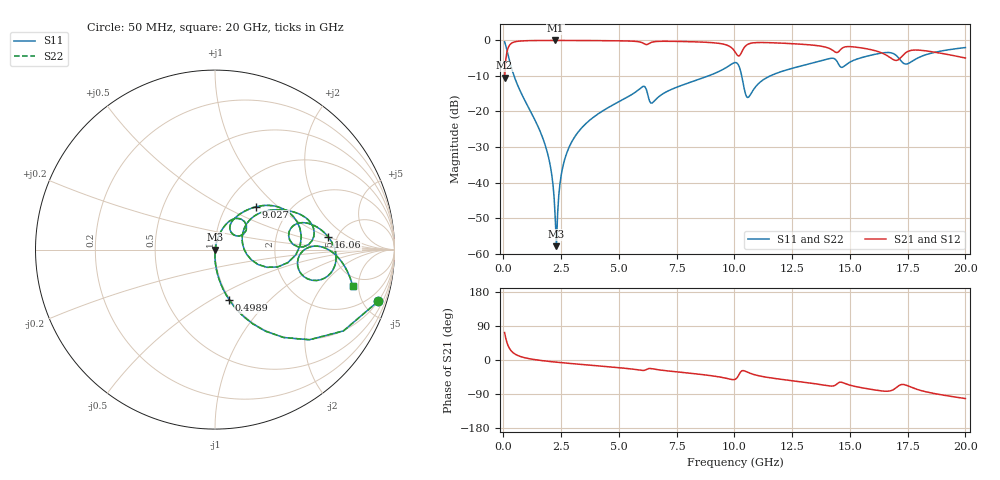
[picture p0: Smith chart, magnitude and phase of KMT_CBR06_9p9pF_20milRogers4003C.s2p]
! Data measured by Modelithics Inc. support@modelithics.com 813-866-6335
! KEMET CBR0603 9.9pF, Pad Width= 0.851mm, Pad Length= 0.64mm, Pad Gap= 0.62mm, 20mil Rogers 4003C substrate Data, January 2022
# hz S ma R 50
! 2 Port Network Data from SP1.SP block
! freq  magS11  angS11  magS21  angS21  magS12  angS12  magS22  angS22
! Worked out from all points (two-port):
!   401 points, 50 MHz to 20 GHz, reference 50 ohm
!   highest |S21| = -0.01 dB at 2.244 GHz (marker M1); lowest = -10.5 dB at 50 MHz (marker M2)
!   |S21| within 3 dB of the highest: 161.2 MHz to 10.01 GHz (9.844 GHz wide, 194 % of centre); 10.33 GHz to 14.31 GHz (3.972 GHz wide, 32.2 % of centre)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
!   lowest |S11| = -57.9 dB at 2.294 GHz (marker M3), VSWR 1.00, Z = 50.1 + j0.0212 ohm
!   |S11| at or under -10 dB: 459.4 MHz to 8.868 GHz (8.409 GHz wide, 180 % of centre); 10.31 GHz to 11.55 GHz (1.231 GHz wide, 11.3 % of centre)
!   |S22| runs from -57.9 to -0.4 dB; largest |S21 - S12| = 0
!   S11 on the Smith chart (normalised r, x): 50 MHz: 0.99, -6.33; 498.9 MHz: 0.99, -0.61; 9.027 GHz: 1.37, +0.73; 16.06 GHz: 4.22, +1.01; 20 GHz: 3.86, -4.26
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5e7  0.954 -17.5  0.2993 72.4  0.2993 72.4  0.954 -17.5
2.99375e8  0.4637 -63.0  0.8854 26.9  0.8854 26.9  0.4637 -63.0
4.98875e8  0.2913 -74.2  0.9559 15.7  0.9559 15.7  0.2913 -74.2
1.8455e9  0.03064 -90.8  0.9983 -2.8  0.9983 -2.8  0.03064 -90.8
2.045e9  0.01604 -90.0  0.9986 -4.2  0.9986 -4.2  0.01604 -90.0
2.2445e9  0.003042 -71.9  0.9987 -5.4  0.9987 -5.4  0.003042 -71.9
2.294375e9  0.001273 9.6  0.9987 -5.7  0.9987 -5.7  0.001273 9.6
2.693375e9  0.02349 78.7  0.9983 -8.1  0.9983 -8.1  0.02349 78.7
3.391625e9  0.05901 76.7  0.9966 -11.8  0.9966 -11.8  0.05901 76.7
5.985125e9  0.2194 51.9  0.9352 -27.3  0.9352 -27.3  0.2194 51.9
6.384125e9  0.1314 40.5  0.9335 -22.6  0.9335 -22.6  0.1314 40.5
6.73325e9  0.1623 58.3  0.9704 -26.0  0.9704 -26.0  0.1623 58.3
9.0275e9  0.3313 46.1  0.9304 -41.7  0.9304 -41.7  0.3313 46.1
1.0025e10  0.4879 14.3  0.6928 -51.2  0.6928 -51.2  0.4879 14.3
1.027438e10  0.3617 -15.5  0.6463 -30.9  0.6463 -30.9  0.3617 -15.5
1.057362e10  0.157 10.8  0.8793 -32.3  0.8793 -32.3  0.157 10.8
1.336662e10  0.4793 26.3  0.8596 -61.6  0.8596 -61.6  0.4793 26.3
1.446388e10  0.4932 1.8  0.6779 -61.9  0.6779 -61.9  0.4932 1.8
1.605988e10  0.6348 6.4  0.7215 -78.9  0.7215 -78.9  0.6348 6.4
1.670825e10  0.675 -6.9  0.5831 -81.9  0.5831 -81.9  0.675 -6.9
1.74065e10  0.465 -8.8  0.6674 -65.9  0.6674 -65.9  0.465 -8.8
2e10  0.7938 -14.9  0.565 -101.8  0.565 -101.8  0.7938 -14.9
